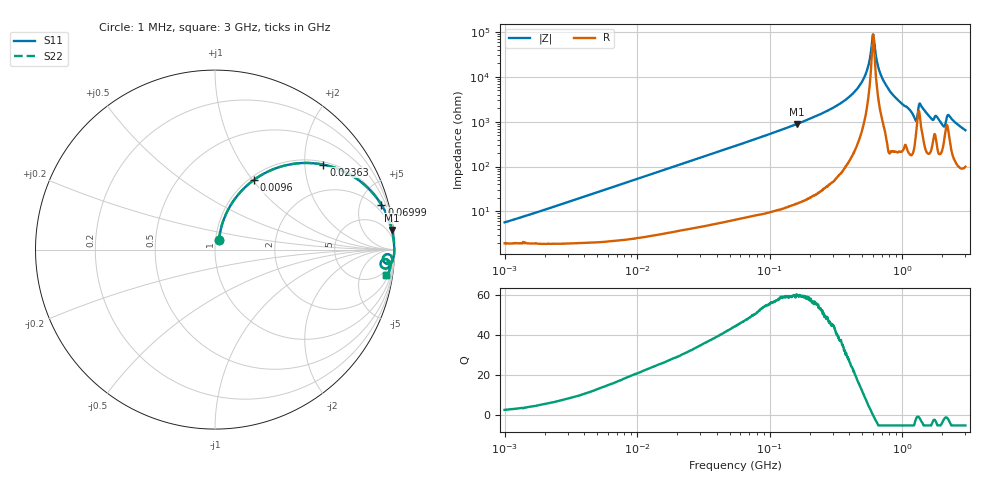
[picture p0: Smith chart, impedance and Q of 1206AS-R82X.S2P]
!s-Parameter Generated by FASTRON Sdn. Bhd.
!FASTRON P/N : 1206AS-R82X
!Keysight Technologies: E4991B_MY54100416_A.01.15
!Date created: Thu Nov 16 13:28:21 2023
!Version  : Rev00 Thu Nov 16 13:28:21 2023
!Data & Calibration Information:
!Freq	S11	S21	S12	S22
!PortZ  Port1:50+j0  Port2:50+j0
!When reading reference impedance value at option line is always used.
! Remarks : This data is being provided solely for informational purposes.
# Hz S dB R 50
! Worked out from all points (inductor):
!   1601 points, 1 MHz to 3 GHz, reference 50 ohm
!   read as one part in series: L = 853 nH near 1.083 MHz
!   highest Q = 59.6 at 161.4 MHz (marker M1), where L = 882 nH
!   self-resonance near 601.9 MHz
!   S11 on the Smith chart (normalised r, x): 1 MHz: 1.04, +0.11; 9.6 MHz: 1.05, +1.02; 23.63 MHz: 1.08, +2.49; 69.99 MHz: 1.15, +7.35; 3 GHz: 3, -13
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1000000  -25.05 67.0  -0.18 -3.0  -0.18 -3.0  -25.05 67.0
3804036  -14.13 73.2  -0.34 -11.3  -0.34 -11.3  -14.13 73.2
9600343  -7.01 60.7  -1.17 -26.5  -1.17 -26.5  -7.01 60.7
1.447069e7  -4.48 51.1  -2.17 -36.6  -2.17 -36.6  -4.48 51.1
2.362996e7  -2.30 38.1  -4.19 -50.1  -4.19 -50.1  -2.30 38.1
5.477226e7  -0.56 19.1  -9.72 -69.6  -9.72 -69.6  -0.56 19.1
6.999185e7  -0.35 15.1  -11.67 -73.7  -11.67 -73.7  -0.35 15.1
1.614254e8  -0.07 6.4  -19.10 -82.7  -19.10 -82.7  -0.07 6.4
2.083556e8  -0.04 4.7  -21.72 -84.3  -21.72 -84.3  -0.04 4.7
3.385367e8  -0.02 2.3  -28.03 -86.2  -28.03 -86.2  -0.02 2.3
4.548043e8  -0.01 1.1  -34.50 -85.8  -34.50 -85.8  -0.01 1.1
5.337858e8  -0.01 0.5  -41.68 -82.2  -41.68 -82.2  -0.01 0.5
6.018993e8  -0.01 0.0  -58.86 -11.4  -58.86 -11.4  -0.01 0.0
6.821091e8  -0.01 -0.5  -41.69 81.0  -41.69 81.0  -0.01 -0.5
7.925923e8  -0.01 -1.1  -34.37 86.6  -34.37 86.6  -0.01 -1.1
1.243477e9  -0.21 -4.6  -21.68 70.5  -21.68 70.5  -0.21 -4.6
1.381259e9  -0.14 -2.2  -27.57 66.2  -27.57 66.2  -0.14 -2.2
1.662201e9  -0.18 -4.7  -21.48 73.3  -21.48 73.3  -0.18 -4.7
1.818868e9  -0.18 -4.1  -22.56 71.6  -22.56 71.6  -0.18 -4.1
2.040726e9  -0.43 -6.4  -18.52 62.6  -18.52 62.6  -0.43 -6.4
2.255531e9  -0.24 -3.8  -23.02 65.3  -23.02 65.3  -0.24 -3.8
3e9  -0.30 -8.5  -16.51 72.7  -16.51 72.7  -0.30 -8.5
